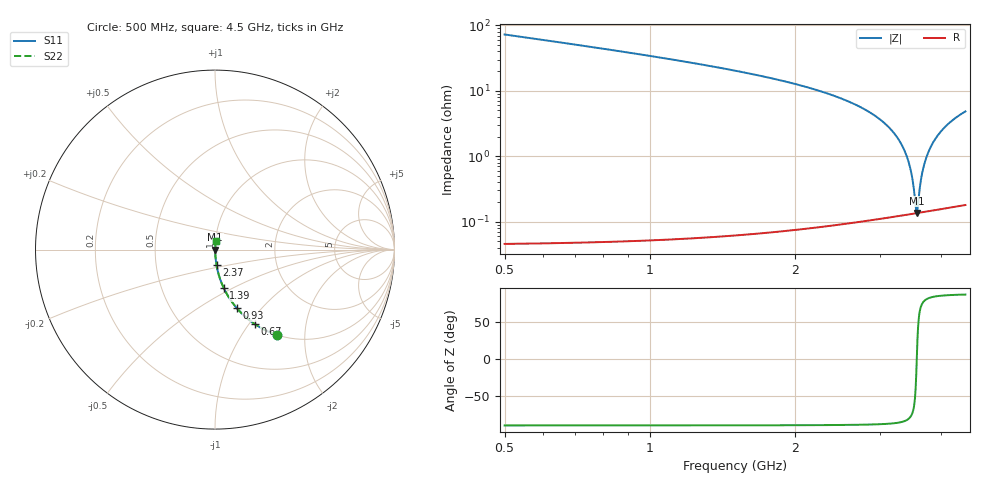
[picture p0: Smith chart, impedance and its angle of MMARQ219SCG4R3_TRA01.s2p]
! MMARQ219SCG4R3_TRA01  S-PARAMETER MODEL  ( General Type )
! Model Generated by TAIYO YUDEN Corporation (http://www.ty-top.com)
! Version 1.0
! TAIYO YUDEN Control No. 180601
! Copyright(c) 2018 TAIYO YUDEN CO.,LTD. All Rights Reserved.
! Product Description (link to TY-COMPAS)
! https://ds.yuden.co.jp/TYCOMPAS/or/detail?pn=MMARQ219SCG4R3BTRA01&u=M
! Products Name : Multilayer Ceramic Capacitors
! Characteristics :
!  Capacitance : 4.3 pF , Rated Voltage : 250V , TCC : CG / C0G
!  Case Size : 2.0 x 1.25 / 0.079 x 0.049 [mm/inch] , Thickness : 0.85 / 0.033 [mm/inch]
!  (Conditions: Temperature = 25 degC , DC Bias Current/Voltage = 0A / 0V)
! External Node Assignments :
!  1  o---| |---o  2
! GND o---------o GND
! Frequency Range : 500MHz  -  4500MHz  [ 401 STEP ]
# MHz S RI R 50
! Freq[MHz].  S11 Real  S11 Imag  S21 Real  S21 Imag  S12 Real  S12 Imag  S22 Real  S22 Imag
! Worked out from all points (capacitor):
!   401 points, 500 MHz to 4.5 GHz, reference 50 ohm
!   read as one part in series: C = 4.3 pF near 520 MHz
!   lowest |Z| = 135 mohm at 3.57 GHz (marker M1)
!   series resonance near 3.569 GHz, so ESL is about 460 pH
!   S11 on the Smith chart (normalised r, x): 500 MHz: 1.00, -1.45; 670 MHz: 1.00, -1.07; 930 MHz: 1.00, -0.74; 1.39 GHz: 1.00, -0.45; 2.37 GHz: 1.00, -0.17; 4.5 GHz: 1.00, +0.10
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500  0.3453 -0.4751  0.6547 0.4751  0.6547 0.4751  0.3453 -0.4751
670  0.2216 -0.4148  0.7784 0.4148  0.7784 0.4148  0.2216 -0.4148
930  0.1214 -0.3259  0.8786 0.3259  0.8786 0.3259  0.1214 -0.3259
1170  0.0743 -0.2613  0.9257 0.2613  0.9257 0.2613  0.0743 -0.2613
1390  0.0491 -0.2147  0.9509 0.2147  0.9509 0.2147  0.0491 -0.2147
1840  0.022 -0.1443  0.978 0.1443  0.978 0.1443  0.022 -0.1443
2370  0.00839 -0.0864  0.9916 0.0864  0.9916 0.0864  0.00839 -0.0864
2500  0.00654 -0.0748  0.9935 0.0748  0.9935 0.0748  0.00654 -0.0748
2890  0.00298 -0.0438  0.997 0.0438  0.997 0.0438  0.00298 -0.0438
3170  0.00177 -0.0245  0.9982 0.0245  0.9982 0.0245  0.00177 -0.0245
3310  0.00147 -0.0156  0.9985 0.0156  0.9985 0.0156  0.00147 -0.0156
3420  0.00136 -0.00879  0.9986 0.00879  0.9986 0.00879  0.00136 -0.00879
3490  0.00133 -0.0046  0.9987 0.0046  0.9987 0.0046  0.00133 -0.0046
3550  0.00134 -0.00108  0.9987 0.00108  0.9987 0.00108  0.00134 -0.00108
3570  0.00134 7.58e-05  0.9987 -7.58e-05  0.9987 -7.58e-05  0.00134 7.58e-05
3590  0.00136 0.00123  0.9986 -0.00123  0.9986 -0.00123  0.00136 0.00123
3640  0.00139 0.00408  0.9986 -0.00408  0.9986 -0.00408  0.00139 0.00408
3680  0.00144 0.00634  0.9986 -0.00634  0.9986 -0.00634  0.00144 0.00634
3750  0.00153 0.0102  0.9985 -0.0102  0.9985 -0.0102  0.00153 0.0102
3840  0.0017 0.0151  0.9983 -0.0151  0.9983 -0.0151  0.0017 0.0151
4110  0.00245 0.0292  0.9975 -0.0292  0.9975 -0.0292  0.00245 0.0292
4500  0.00411 0.0481  0.9959 -0.0481  0.9959 -0.0481  0.00411 0.0481
